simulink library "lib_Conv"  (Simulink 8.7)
settings: Solver=ode45  StartTime=0.0  StopTime=10.0  RelTol=1e-3
undefined symbols (not defined in the file or in its folder): b0bit, b1bit, b2bit, b3bit, b4bit, b5bit, b6bit, b7bit, bit, Bitnr, hi, lo, maxFader
libraries: lib_Conv x8, simulink x1

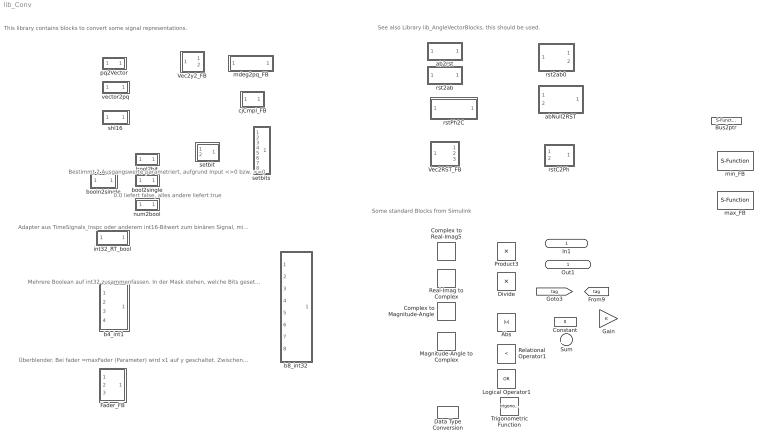
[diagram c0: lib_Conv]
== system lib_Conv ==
  note: Some standard Blocks from Simulink
  note: Mehrere Boolean auf int32 zusammenfassen. In der Mask stehen, welche Bits gesetzt werden. Default ist 0..3 bzw. 0..7, lässt sich ändern.
  note: Überblender. Bei fader =maxFader (Parameter) wird x1 auf y geschaltet. Zwischen diesen Werten überblenden.
  note: Adapter aus TimeSignals_Inspc oder anderem int16-Bitwert zum binären Signal, mit Angabe Bit-Nummer als Parameter. Einschließlich Rate-Transition, Ausgang kann in TstepHw direkt verwendet werden.
  note: See also Library lib_AngleVectorBlocks, this should be used.
  note: This library contains blocks to convert some signal representations.
  note: Bestimmt 2 Ausgangswerte parametriert, aufgrund Input <>0 bzw. >=0
  note: 0.0 liefert false, alles andere liefert true
  In1 : Inport  OutDataTypeStr=single  PortDimensions=1
  Abs : Abs
  Bus2ptr : S-Function  FunctionName=Bus2ptr_mex  SFunctionDeploymentMode=off  EnableBusSupport=off
  Complex to Magnitude-Angle : ComplexToMagnitudeAngle
  Complex to Real-Imag5 : ComplexToRealImag
  Constant : Constant  Value=0  OutDataTypeStr=single
  Data Type Conversion : DataTypeConversion  OutDataTypeStr=int32
  Divide : Product  Inputs=*/
  Fader_FB : Subsystem
  Gain : Gain
  Logical Operator1 : Logic  Operator=OR  IconShape=distinctive  AllPortsSameDT=off  OutDataTypeStr=boolean
  Magnitude-Angle to Complex : MagnitudeAngleToComplex
  Product3 : Product
  Real-Imag to Complex : RealImagToComplex
  Relational Operator1 : RelationalOperator  Operator=<  OutDataTypeStr=boolean
  Sum : Sum  Inputs=|++
  Trigonometric Function : Trigonometry
  Vec2RST_FB : Subsystem
  Vec2y2_FB : Subsystem
  ab2rst : Subsystem
  abNull2RST : Subsystem
  b4_int1 : Subsystem
  b8_int32 : Subsystem
  bool2bit : Subsystem
  bool2single : Subsystem
  booln2single : Subsystem
  cjCmpl_FB : Subsystem
  int32_RT_bool : Subsystem
  max_FB : S-Function  FunctionName=max_FB  SFunctionDeploymentMode=off  EnableBusSupport=off
  mdeg2pq_FB : Subsystem
  min_FB : S-Function  FunctionName=min_FB_mex  SFunctionDeploymentMode=off  EnableBusSupport=off
  num2bool : Subsystem
  pq2Vector : Subsystem
  rst2ab : Subsystem
  rst2ab0 : Subsystem
  rstC2Ph : Subsystem
  rstPh2C : Subsystem
  setbit : Subsystem
  setbits : Subsystem
  shl16 : Subsystem  TreatAsAtomicUnit=on
  vector2pq : Subsystem
  Out1 : Outport  OutDataTypeStr=single  PortDimensions=1

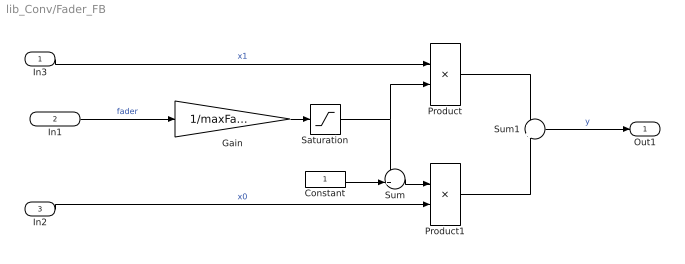
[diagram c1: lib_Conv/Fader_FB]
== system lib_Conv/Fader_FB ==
  In3 : Inport  OutDataTypeStr=single
  In1 : Inport  Port=2  OutDataTypeStr=single
  In2 : Inport  Port=3  OutDataTypeStr=single
  Constant : Constant  OutDataTypeStr=single
  Gain : Gain  Gain=1/maxFader
  Product : Product
  Product1 : Product
  Saturation : Saturate  UpperLimit=1  LowerLimit=0  ZeroCross=off
  Sum : Sum  Inputs=-+|
  Sum1 : Sum  Inputs=+|+
  Out1 : Outport  OutDataTypeStr=single
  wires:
  In1/1 -> Gain/1  "fader"
  Gain/1 -> Saturation/1
  Saturation/1 -> Product/2, Sum/1
  Constant/1 -> Sum/2
  Sum/1 -> Product1/1
  In2/1 -> Product1/2  "x0"
  In3/1 -> Product/1  "x1"
  Product/1 -> Sum1/1
  Product1/1 -> Sum1/2
  Sum1/1 -> Out1/1  "y"

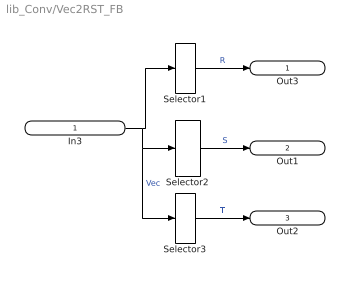
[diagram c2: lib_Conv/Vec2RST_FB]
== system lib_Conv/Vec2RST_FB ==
  In3 : Inport  PortDimensions=3
  Selector1 : Selector  InputPortWidth=3  IndexOptions=Index vector (dialog)  Indices=[1]  OutputSizes=1
  Selector2 : Selector  InputPortWidth=3  IndexOptions=Index vector (dialog)  Indices=[2]  OutputSizes=1
  Selector3 : Selector  InputPortWidth=3  IndexOptions=Index vector (dialog)  Indices=[3]  OutputSizes=1
  Out3 : Outport  PortDimensions=1
  Out1 : Outport  Port=2  PortDimensions=1
  Out2 : Outport  Port=3  PortDimensions=1
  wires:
  In3/1 -> Selector3/1, Selector2/1, Selector1/1  "Vec"
  Selector1/1 -> Out3/1  "R"
  Selector2/1 -> Out1/1  "S"
  Selector3/1 -> Out2/1  "T"

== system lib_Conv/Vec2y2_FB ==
  In1 : Inport  PortDimensions=2
  Selector : Selector  IndexMode=Zero-based  InputPortWidth=2  IndexOptions=Index vector (dialog)  Indices=[0]  OutputSizes=1
  Selector1 : Selector  IndexMode=Zero-based  InputPortWidth=2  IndexOptions=Index vector (dialog)  Indices=[1]  OutputSizes=1
  Out1 : Outport
  Out2 : Outport  Port=2
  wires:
  Selector1/1 -> Out2/1  "y2"
  In1/1 -> Selector1/1, Selector/1
  Selector/1 -> Out1/1  "y1"

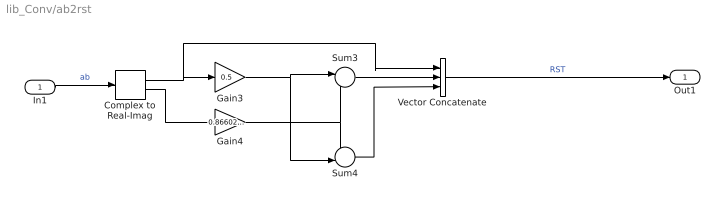
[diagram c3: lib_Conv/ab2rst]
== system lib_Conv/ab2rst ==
  In1 : Inport  OutDataTypeStr=single
  Complex to Real-Imag : ComplexToRealImag
  Gain3 : Gain  Gain=0.5
  Gain4 : Gain  Gain=0.86602540  OutDataTypeStr=single
  Sum3 : Sum  Inputs=|-+
  Sum4 : Sum  Inputs=--|
  Vector Concatenate : Concatenate  NumInputs=3
  Out1 : Outport
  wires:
  Vector Concatenate/1 -> Out1/1  "RST"
  In1/1 -> Complex to Real-Imag/1  "ab"
  Complex to Real-Imag/1 -> Vector Concatenate/1, Gain3/1
  Complex to Real-Imag/2 -> Gain4/1
  Gain3/1 -> Sum4/2, Sum3/1
  Gain4/1 -> Sum3/2, Sum4/1
  Sum3/1 -> Vector Concatenate/2
  Sum4/1 -> Vector Concatenate/3

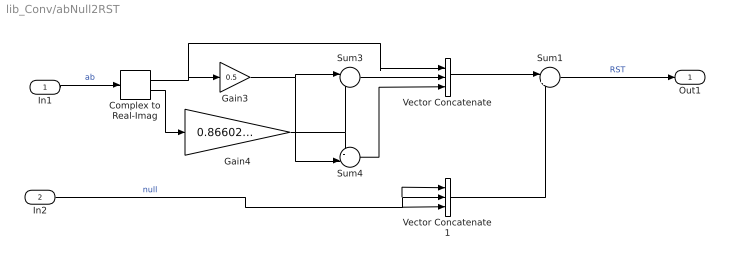
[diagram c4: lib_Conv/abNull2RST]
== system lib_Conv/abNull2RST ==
  In1 : Inport  OutDataTypeStr=single  PortDimensions=1
  In2 : Inport  Port=2  OutDataTypeStr=single  PortDimensions=1
  Complex to Real-Imag : ComplexToRealImag
  Gain3 : Gain  Gain=0.5
  Gain4 : Gain  Gain=0.86602540  OutDataTypeStr=single
  Sum1 : Sum  Inputs=|++
  Sum3 : Sum  Inputs=|-+
  Sum4 : Sum  Inputs=--|
  Vector Concatenate : Concatenate  NumInputs=3
  Vector Concatenate1 : Concatenate  NumInputs=3
  Out1 : Outport  PortDimensions=3
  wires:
  Vector Concatenate1/1 -> Sum1/2
  In2/1 -> Vector Concatenate1/3, Vector Concatenate1/2, Vector Concatenate1/1  "null"
  Vector Concatenate/1 -> Sum1/1
  Sum4/1 -> Vector Concatenate/3
  Sum3/1 -> Vector Concatenate/2
  Gain4/1 -> Sum4/1, Sum3/2
  Gain3/1 -> Sum3/1, Sum4/2
  Complex to Real-Imag/2 -> Gain4/1
  Complex to Real-Imag/1 -> Gain3/1, Vector Concatenate/1
  In1/1 -> Complex to Real-Imag/1  "ab"
  Sum1/1 -> Out1/1  "RST"

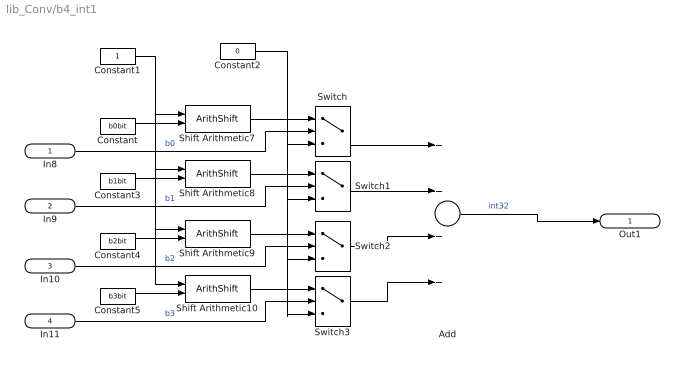
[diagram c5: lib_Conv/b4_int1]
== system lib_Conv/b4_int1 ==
  In8 : Inport  OutDataTypeStr=boolean
  In9 : Inport  Port=2  OutDataTypeStr=boolean
  In10 : Inport  Port=3  OutDataTypeStr=boolean
  In11 : Inport  Port=4  OutDataTypeStr=boolean
  Add : Sum  Inputs=++++
  Constant : Constant  Value=b0bit  OutDataTypeStr=uint32
  Constant1 : Constant  OutDataTypeStr=uint32
  Constant2 : Constant  Value=0  OutDataTypeStr=uint32
  Constant3 : Constant  Value=b1bit  OutDataTypeStr=uint32
  Constant4 : Constant  Value=b2bit  OutDataTypeStr=uint32
  Constant5 : Constant  Value=b3bit  OutDataTypeStr=uint32
  Shift Arithmetic{7..10} (4 alike) : ArithShift  BitShiftNumberSource=Input port  BitShiftNumber=6  BitShiftDirection=Left
  Switch{,1..3} (4 alike) : Switch  Criteria=u2 ~= 0  OutDataTypeStr=uint32
  Out1 : Outport  OutDataTypeStr=uint32  PortDimensions=1
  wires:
  In8/1 -> Switch/2  "b0"
  Add/1 -> Out1/1  "int32"
  Constant/1 -> Shift Arithmetic7/2
  Shift Arithmetic7/1 -> Switch/1
  Constant1/1 -> Shift Arithmetic10/1, Shift Arithmetic9/1, Shift Arithmetic8/1, Shift Arithmetic7/1
  Constant2/1 -> Switch1/3, Switch3/3, Switch2/3, Switch/3
  In9/1 -> Switch1/2  "b1"
  Constant3/1 -> Shift Arithmetic8/2
  Shift Arithmetic8/1 -> Switch1/1
  In10/1 -> Switch2/2  "b2"
  Constant4/1 -> Shift Arithmetic9/2
  Shift Arithmetic9/1 -> Switch2/1
  In11/1 -> Switch3/2  "b3"
  Constant5/1 -> Shift Arithmetic10/2
  Shift Arithmetic10/1 -> Switch3/1
  Switch/1 -> Add/1
  Switch1/1 -> Add/2
  Switch2/1 -> Add/3
  Switch3/1 -> Add/4

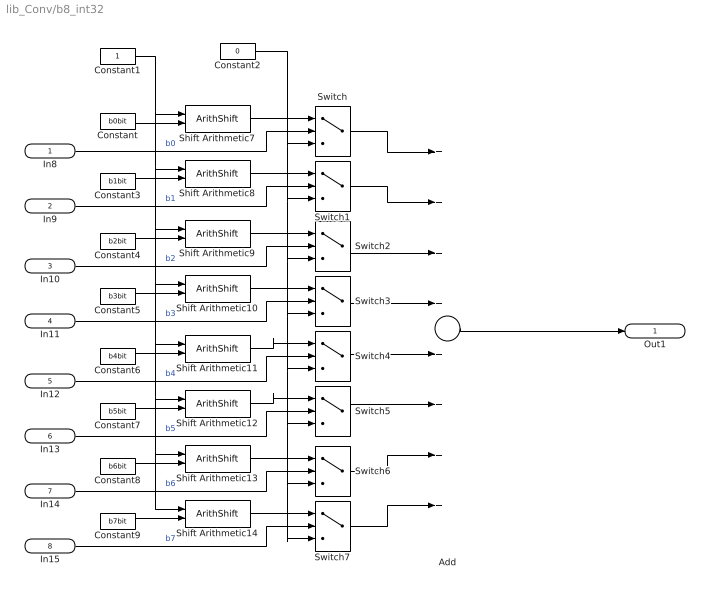
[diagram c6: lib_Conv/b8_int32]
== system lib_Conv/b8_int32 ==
  In8 : Inport  OutDataTypeStr=boolean
  In9 : Inport  Port=2  OutDataTypeStr=boolean
  In10 : Inport  Port=3  OutDataTypeStr=boolean
  In11 : Inport  Port=4  OutDataTypeStr=boolean
  In12 : Inport  Port=5  OutDataTypeStr=boolean
  In13 : Inport  Port=6  OutDataTypeStr=boolean
  In14 : Inport  Port=7  OutDataTypeStr=boolean
  In15 : Inport  Port=8  OutDataTypeStr=boolean
  Add : Sum  Inputs=++++++++
  Constant : Constant  Value=b0bit  OutDataTypeStr=uint32
  Constant1 : Constant  OutDataTypeStr=uint32
  Constant2 : Constant  Value=0  OutDataTypeStr=uint32
  Constant3 : Constant  Value=b1bit  OutDataTypeStr=uint32
  Constant4 : Constant  Value=b2bit  OutDataTypeStr=uint32
  Constant5 : Constant  Value=b3bit  OutDataTypeStr=uint32
  Constant6 : Constant  Value=b4bit  OutDataTypeStr=uint32
  Constant7 : Constant  Value=b5bit  OutDataTypeStr=uint32
  Constant8 : Constant  Value=b6bit  OutDataTypeStr=uint32
  Constant9 : Constant  Value=b7bit  OutDataTypeStr=uint32
  Shift Arithmetic{7..14} (8 alike) : ArithShift  BitShiftNumberSource=Input port  BitShiftNumber=6  BitShiftDirection=Left
  Switch{,1..7} (8 alike) : Switch  Criteria=u2 ~= 0  OutDataTypeStr=uint32
  Out1 : Outport  OutDataTypeStr=uint32  PortDimensions=1
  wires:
  In8/1 -> Switch/2  "b0"
  Constant/1 -> Shift Arithmetic7/2
  Shift Arithmetic7/1 -> Switch/1
  Constant1/1 -> Shift Arithmetic14/1, Shift Arithmetic13/1, Shift Arithmetic12/1, Shift Arithmetic11/1, Shift Arithmetic10/1, Shift Arithmetic9/1, Shift Arithmetic8/1, Shift Arithmetic7/1
  Constant2/1 -> Switch/3, Switch1/3, Switch2/3, Switch3/3, Switch6/3, Switch7/3, Switch5/3, Switch4/3
  In9/1 -> Switch1/2  "b1"
  Constant3/1 -> Shift Arithmetic8/2
  Shift Arithmetic8/1 -> Switch1/1
  In10/1 -> Switch2/2  "b2"
  Constant4/1 -> Shift Arithmetic9/2
  Shift Arithmetic9/1 -> Switch2/1
  In11/1 -> Switch3/2  "b3"
  Constant5/1 -> Shift Arithmetic10/2
  Shift Arithmetic10/1 -> Switch3/1
  In12/1 -> Switch4/2  "b4"
  Constant6/1 -> Shift Arithmetic11/2
  Shift Arithmetic11/1 -> Switch4/1
  In13/1 -> Switch5/2  "b5"
  Constant7/1 -> Shift Arithmetic12/2
  Shift Arithmetic12/1 -> Switch5/1
  In14/1 -> Switch6/2  "b6"
  Constant8/1 -> Shift Arithmetic13/2
  Shift Arithmetic13/1 -> Switch6/1
  In15/1 -> Switch7/2  "b7"
  Constant9/1 -> Shift Arithmetic14/2
  Shift Arithmetic14/1 -> Switch7/1
  Switch/1 -> Add/1
  Switch1/1 -> Add/2
  Switch2/1 -> Add/3
  Switch3/1 -> Add/4
  Switch7/1 -> Add/8
  Switch6/1 -> Add/7
  Switch5/1 -> Add/6
  Switch4/1 -> Add/5
  Add/1 -> Out1/1

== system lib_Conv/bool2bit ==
  b : Inport
  Constant : Constant  Value=bit  OutDataTypeStr=int32
  Constant1 : Constant  Value=0  OutDataTypeStr=int32
  Switch : Switch  Criteria=u2 ~= 0  OutDataTypeStr=int32
  y : Outport  OutDataTypeStr=int32
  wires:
  Switch/1 -> y/1
  b/1 -> Switch/2  "b"
  Constant1/1 -> Switch/3
  Constant/1 -> Switch/1

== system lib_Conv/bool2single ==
  b : Inport
  Constant : Constant  Value=hi  OutDataTypeStr=single
  Constant1 : Constant  Value=lo  OutDataTypeStr=single
  Switch : Switch  Criteria=u2 ~= 0
  y : Outport  OutDataTypeStr=single
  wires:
  Constant/1 -> Switch/1
  Constant1/1 -> Switch/3
  b/1 -> Switch/2  "b"
  Switch/1 -> y/1

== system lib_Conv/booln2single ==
  b : Inport
  Constant : Constant  Value=hi  OutDataTypeStr=single
  Constant1 : Constant  Value=lo  OutDataTypeStr=single
  Switch : Switch
  y : Outport
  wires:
  Constant/1 -> Switch/1
  Constant1/1 -> Switch/3
  b/1 -> Switch/2  "b"
  Switch/1 -> y/1

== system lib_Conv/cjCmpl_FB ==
  In1 : Inport  OutDataTypeStr=single
  Complex to Real-Imag : ComplexToRealImag
  Gain : Gain  Gain=-1
  Real-Imag to Complex : RealImagToComplex
  Out1 : Outport  OutDataTypeStr=single
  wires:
  In1/1 -> Complex to Real-Imag/1  "xpq"
  Complex to Real-Imag/1 -> Real-Imag to Complex/1
  Real-Imag to Complex/1 -> Out1/1  "nq"
  Complex to Real-Imag/2 -> Gain/1
  Gain/1 -> Real-Imag to Complex/2

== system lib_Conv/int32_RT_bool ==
  In1 : Inport  OutDataTypeStr=int16
  Bitwise Operator : simulink/Logic and Bit Operations/Bitwise Operator  logicop=AND  UseBitMask=on  BitMask=bitshift(1,Bitnr)  BitMaskRealWorld=Stored Integer
  Data Type Conversion : DataTypeConversion  OutDataTypeStr=boolean
  Rate Transition7 : RateTransition  OutPortSampleTime=TstepHw
  Out1 : Outport  OutDataTypeStr=boolean
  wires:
  Data Type Conversion/1 -> Rate Transition7/1
  Bitwise Operator/1 -> Data Type Conversion/1
  In1/1 -> Bitwise Operator/1  "x16_RT"
  Rate Transition7/1 -> Out1/1  "bin"

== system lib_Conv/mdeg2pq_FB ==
  In1 : Inport  PortDimensions=2
  Gain : Gain  Gain=pi/180
  Magnitude-Angle to Complex3 : MagnitudeAngleToComplex
  Selector : Selector  IndexMode=Zero-based  InputPortWidth=2  IndexOptions=Index vector (dialog)  Indices=[0]  OutputSizes=1
  Selector1 : Selector  IndexMode=Zero-based  InputPortWidth=2  IndexOptions=Index vector (dialog)  Indices=[1]  OutputSizes=1
  Out1 : Outport
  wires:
  Selector1/1 -> Gain/1  "y2"
  In1/1 -> Selector1/1, Selector/1  "mdeg"
  Magnitude-Angle to Complex3/1 -> Out1/1  "pq"
  Selector/1 -> Magnitude-Angle to Complex3/1  "y1"
  Gain/1 -> Magnitude-Angle to Complex3/2

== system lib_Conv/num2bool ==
  x : Inport
  Constant1 : Constant  Value=0  OutDataTypeStr=single
  Relational Operator : RelationalOperator  Operator=~=  OutDataTypeStr=boolean
  b : Outport
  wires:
  Relational Operator/1 -> b/1
  Constant1/1 -> Relational Operator/2
  x/1 -> Relational Operator/1

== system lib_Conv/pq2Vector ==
  In1 : Inport  PortDimensions=1
  Complex to Real-Imag : ComplexToRealImag
  Vector Concatenate : Concatenate
  Out1 : Outport  PortDimensions=2
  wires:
  Complex to Real-Imag/1 -> Vector Concatenate/1
  Complex to Real-Imag/2 -> Vector Concatenate/2
  In1/1 -> Complex to Real-Imag/1
  Vector Concatenate/1 -> Out1/1  "pqV"

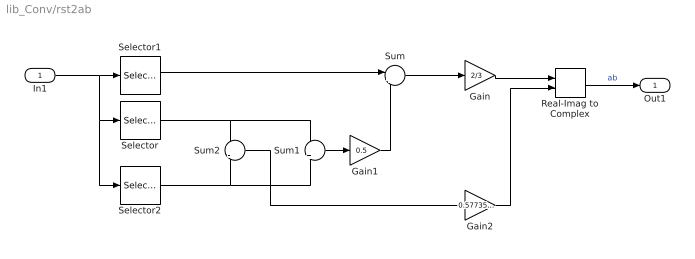
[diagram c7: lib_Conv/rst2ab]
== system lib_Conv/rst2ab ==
  In1 : Inport
  Gain : Gain  Gain=2/3
  Gain1 : Gain  Gain=0.5
  Gain2 : Gain  Gain=0.5773502692
  Real-Imag to Complex : RealImagToComplex
  Selector : Selector  InputPortWidth=3  IndexOptions=Index vector (dialog)  Indices=[2]  OutputSizes=1
  Selector1 : Selector  InputPortWidth=3  IndexOptions=Index vector (dialog)  Indices=[1]  OutputSizes=1
  Selector2 : Selector  InputPortWidth=3  IndexOptions=Index vector (dialog)  Indices=[3]  OutputSizes=1
  Sum : Sum  Inputs=|+-
  Sum1 : Sum  Inputs=+|+
  Sum2 : Sum  Inputs=+|-
  Out1 : Outport
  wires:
  Gain/1 -> Real-Imag to Complex/1
  Sum2/1 -> Gain2/1
  Gain2/1 -> Real-Imag to Complex/2
  Real-Imag to Complex/1 -> Out1/1  "ab"
  In1/1 -> Selector/1, Selector2/1, Selector1/1
  Selector2/1 -> Sum2/2, Sum1/2
  Selector1/1 -> Sum/1
  Gain1/1 -> Sum/2
  Sum1/1 -> Gain1/1
  Selector/1 -> Sum2/1, Sum1/1
  Sum/1 -> Gain/1

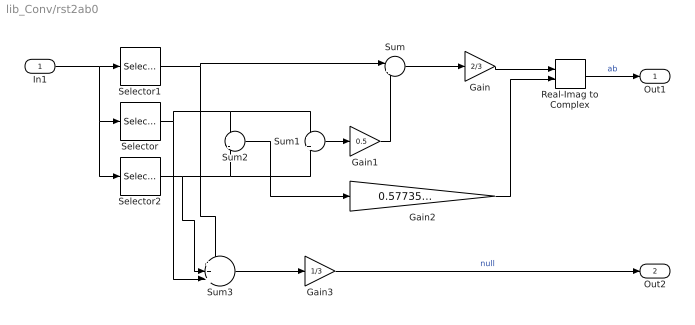
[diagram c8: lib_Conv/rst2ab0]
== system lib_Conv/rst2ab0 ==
  In1 : Inport
  Gain : Gain  Gain=2/3
  Gain1 : Gain  Gain=0.5
  Gain2 : Gain  Gain=0.5773502692
  Gain3 : Gain  Gain=1/3
  Real-Imag to Complex : RealImagToComplex
  Selector : Selector  InputPortWidth=3  IndexOptions=Index vector (dialog)  Indices=[2]  OutputSizes=1
  Selector1 : Selector  InputPortWidth=3  IndexOptions=Index vector (dialog)  Indices=[1]  OutputSizes=1
  Selector2 : Selector  InputPortWidth=3  IndexOptions=Index vector (dialog)  Indices=[3]  OutputSizes=1
  Sum : Sum  Inputs=|+-
  Sum1 : Sum  Inputs=+|+
  Sum2 : Sum  Inputs=+|-
  Sum3 : Sum  Inputs=+++||
  Out1 : Outport
  Out2 : Outport  Port=2
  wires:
  Gain3/1 -> Out2/1  "null"
  Sum3/1 -> Gain3/1
  Sum/1 -> Gain/1
  Selector/1 -> Sum3/3, Sum1/1, Sum2/1
  Sum1/1 -> Gain1/1
  Gain1/1 -> Sum/2
  Selector1/1 -> Sum/1, Sum3/1
  Selector2/1 -> Sum1/2, Sum2/2, Sum3/2
  In1/1 -> Selector1/1, Selector2/1, Selector/1
  Real-Imag to Complex/1 -> Out1/1  "ab"
  Gain2/1 -> Real-Imag to Complex/2
  Sum2/1 -> Gain2/1
  Gain/1 -> Real-Imag to Complex/1

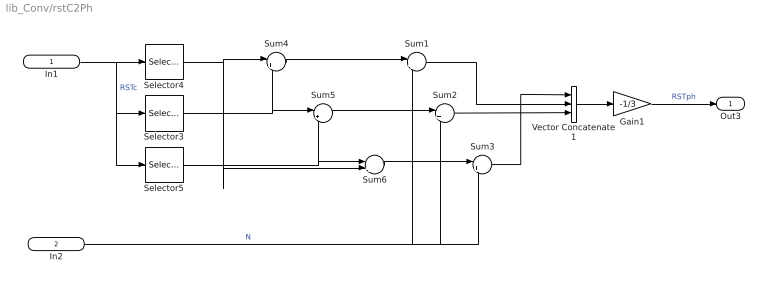
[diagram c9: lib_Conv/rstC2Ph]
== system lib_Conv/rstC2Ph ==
  In1 : Inport
  In2 : Inport  Port=2
  Gain1 : Gain  Gain=-1/3
  Selector3 : Selector  InputPortWidth=3  IndexOptions=Index vector (dialog)  Indices=[2]  OutputSizes=1
  Selector4 : Selector  InputPortWidth=3  IndexOptions=Index vector (dialog)  Indices=[1]  OutputSizes=1
  Selector5 : Selector  InputPortWidth=3  IndexOptions=Index vector (dialog)  Indices=[3]  OutputSizes=1
  Sum{1..6} (6 alike) : Sum  Inputs=|+-
  Vector Concatenate1 : Concatenate  NumInputs=3
  Out3 : Outport
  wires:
  In1/1 -> Selector4/1, Selector3/1, Selector5/1  "RSTc"
  Sum3/1 -> Vector Concatenate1/1
  Sum2/1 -> Vector Concatenate1/3
  Selector5/1 -> Sum6/1, Sum5/2
  Selector3/1 -> Sum5/1, Sum4/2
  Sum1/1 -> Vector Concatenate1/2
  Selector4/1 -> Sum4/1, Sum6/2
  Vector Concatenate1/1 -> Gain1/1
  Gain1/1 -> Out3/1  "RSTph"
  Sum4/1 -> Sum1/1
  Sum6/1 -> Sum3/1
  Sum5/1 -> Sum2/1
  In2/1 -> Sum3/2, Sum2/2, Sum1/2  "N"

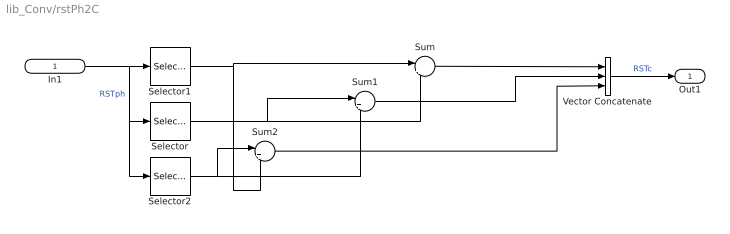
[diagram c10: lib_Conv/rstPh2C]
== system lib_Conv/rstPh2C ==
  In1 : Inport
  Selector : Selector  InputPortWidth=3  IndexOptions=Index vector (dialog)  Indices=[2]  OutputSizes=1
  Selector1 : Selector  InputPortWidth=3  IndexOptions=Index vector (dialog)  Indices=[1]  OutputSizes=1
  Selector2 : Selector  InputPortWidth=3  IndexOptions=Index vector (dialog)  Indices=[3]  OutputSizes=1
  Sum : Sum  Inputs=|+-
  Sum1 : Sum  Inputs=|+-
  Sum2 : Sum  Inputs=|+-
  Vector Concatenate : Concatenate  NumInputs=3
  Out1 : Outport
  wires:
  Vector Concatenate/1 -> Out1/1  "RSTc"
  In1/1 -> Selector/1, Selector2/1, Selector1/1  "RSTph"
  Selector1/1 -> Sum2/2, Sum/1
  Sum/1 -> Vector Concatenate/1
  Selector/1 -> Sum/2, Sum1/1
  Selector2/1 -> Sum1/2, Sum2/1
  Sum1/1 -> Vector Concatenate/2
  Sum2/1 -> Vector Concatenate/3

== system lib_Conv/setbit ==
  b : Inport
  x : Inport  Port=2  OutDataTypeStr=int32
  Constant : Constant  Value=bit  OutDataTypeStr=int32
  Constant1 : Constant  Value=0  OutDataTypeStr=int32
  Sum : Sum  Inputs=|++
  Switch : Switch  Criteria=u2 ~= 0  OutDataTypeStr=int32
  y : Outport  OutDataTypeStr=int32
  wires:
  Constant/1 -> Switch/1
  Constant1/1 -> Switch/3
  b/1 -> Switch/2  "b"
  Sum/1 -> y/1
  Switch/1 -> Sum/1
  x/1 -> Sum/2  "x"

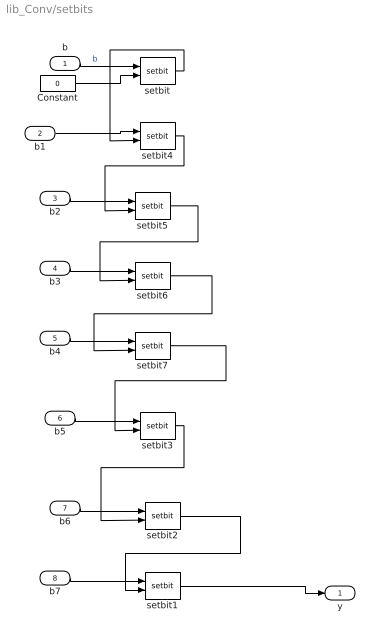
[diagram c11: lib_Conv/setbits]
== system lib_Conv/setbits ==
  b : Inport
  b1 : Inport  Port=2
  b2 : Inport  Port=3
  b3 : Inport  Port=4
  b4 : Inport  Port=5
  b5 : Inport  Port=6
  b6 : Inport  Port=7
  b7 : Inport  Port=8
  Constant : Constant  Value=0  OutDataTypeStr=int32
  setbit : lib_Conv/setbit  bit=1
  setbit1 : lib_Conv/setbit  bit=128
  setbit2 : lib_Conv/setbit  bit=64
  setbit3 : lib_Conv/setbit  bit=32
  setbit4 : lib_Conv/setbit  bit=2
  setbit5 : lib_Conv/setbit  bit=4
  setbit6 : lib_Conv/setbit  bit=8
  setbit7 : lib_Conv/setbit  bit=16
  y : Outport
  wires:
  setbit1/1 -> y/1
  b/1 -> setbit/1  "b"
  Constant/1 -> setbit/2
  setbit/1 -> setbit4/2
  setbit4/1 -> setbit5/2
  setbit5/1 -> setbit6/2
  setbit6/1 -> setbit7/2
  setbit7/1 -> setbit3/2
  setbit3/1 -> setbit2/2
  setbit2/1 -> setbit1/2
  b1/1 -> setbit4/1
  b7/1 -> setbit1/1
  b6/1 -> setbit2/1
  b5/1 -> setbit3/1
  b4/1 -> setbit7/1
  b3/1 -> setbit6/1
  b2/1 -> setbit5/1

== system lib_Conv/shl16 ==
  pq : Inport
  Data Type Conversion1 : DataTypeConversion  OutDataTypeStr=int32  RndMeth=Simplest
  Gain2 : Gain  Gain=65536  OutDataTypeStr=int32
  mwi : Outport  OutDataTypeStr=int32
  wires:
  pq/1 -> Data Type Conversion1/1  "i16"
  Gain2/1 -> mwi/1  "i32"
  Data Type Conversion1/1 -> Gain2/1

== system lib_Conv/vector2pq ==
  In1 : Inport  PortDimensions=2
  Real-Imag to Complex : RealImagToComplex
  Selector : Selector  IndexMode=Zero-based  InputPortWidth=2  IndexOptions=Index vector (dialog)  Indices=[0]  OutputSizes=1
  Selector1 : Selector  IndexMode=Zero-based  InputPortWidth=2  IndexOptions=Index vector (dialog)  Indices=[1]  OutputSizes=1
  Out1 : Outport
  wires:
  Selector1/1 -> Real-Imag to Complex/2
  Real-Imag to Complex/1 -> Out1/1  "pq"
  Selector/1 -> Real-Imag to Complex/1
  In1/1 -> Selector1/1, Selector/1
